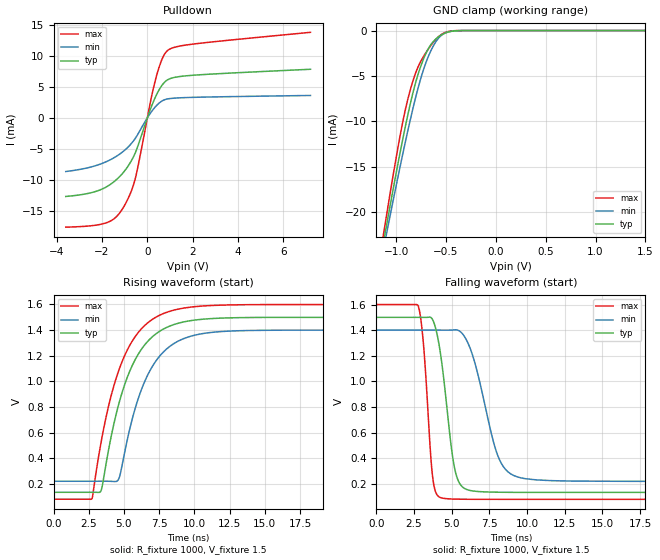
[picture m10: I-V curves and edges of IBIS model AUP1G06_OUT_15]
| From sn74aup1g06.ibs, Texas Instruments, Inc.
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[Model]   AUP1G06_OUT_15
Model_type  Open_drain
Enable   Active-Low
Vref =   1.5
Rref =   1E6
Cref =   30p
Vmeas =   0.75
| variable   typ   min   max
C_comp   1.68pF   1.45pF   1.95pF
| C_pulldown   2.10pF   1.70pF   2.55pF
| C_tri-state   1.68pF   1.45pF   1.95pF
[Temperature Range]   40   100   -40
| Ambient temperature   25   85   -40
[Voltage range]   1.5   1.4   1.6
[Pullup Reference]   1.5   1.5   1.5
[POWER Clamp Reference]   1.5   1.5   1.5
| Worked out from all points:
|   slope of the pulldown table from 0 to 0.225 V, typ, clamps not added: 101 ohm
|   GND clamp passes 1 mA (typ) near -0.61 V on its own axis
|   rising waveform, R_fixture 1000, V_fixture 1.5: 20-80 % time 2.29ns typ, 2.23ns min, 2.33ns max; typ from 0.133 V to 1.5 V
|   falling waveform, R_fixture 1000, V_fixture 1.5: 20-80 % time 824ps typ, 1.46ns min, 510ps max; typ from 1.5 V to 0.133 V
[GND Clamp]
| AUP1G06_OUT_15
|   Voltage   I(typ)   I(min)   I(max)
-3.6V     -193.5mA   -179.7mA   -210.2mA
-1.13V    -23.52mA   -24.27mA   -22.65mA
-1.105V   -21.98mA   -22.86mA   -20.94mA
-1.085V   -20.77mA   -21.75mA   -19.58mA
-950mV    -12.87mA   -14.45mA   -10.98mA
-850mV    -7.682mA   -9.442mA   -6.214mA
-790mV    -5.17mA    -6.745mA   -4.259mA
-720mV    -2.981mA   -4.114mA   -2.762mA
-650mV    -1.523mA   -2.183mA   -1.616mA
-580mV    -733.4uA   -904.6uA   -734uA
-390mV    -21.99uA   -24.69uA   -8.299uA
1.5V      133.6pA    590.3pA    26.39pA
[Pulldown]
| AUP1G06_OUT_15
|   Voltage   I(typ)   I(min)   I(max)
-3.6V     -12.64mA   -8.632mA   -17.58mA
-1.79V    -11.07mA   -7.008mA   -16.85mA
-1.38V    -9.983mA   -6.211mA   -15.95mA
-1.025V   -8.629mA   -5.274mA   -14.21mA
-725mV    -7.022mA   -4.203mA   -11.94mA
-525mV    -5.567mA   -3.253mA   -9.657mA
150mV     1.53mA     832.4uA    2.806mA
420mV     3.835mA    2.043mA    6.955mA
670mV     5.357mA    2.767mA    9.628mA
900mV     6.139mA    3.055mA    10.86mA
1.995V    6.857mA    3.303mA    11.87mA
7.2V      7.827mA    3.609mA    13.77mA
[Ramp]
| AUP1G06_OUT_15
| variable   typ   min   max
dV/dt_r   0.82/2.29E-09   0.71/2.23E-09   0.91/2.33E-09
dV/dt_f   0.82/8.28E-10   0.71/1.47E-09   0.91/5.12E-10
R_load = 1000
[Rising Waveform]
| AUP1G06_OUT_15
R_fixture =   1000
C_fixture =   0
L_fixture =   0
V_fixture =   1.5
V_fixture_min = 1.4
V_fixture_max = 1.6
|   Time   V(typ)   V(min)   V(max)
0s        133.1mV    219.3mV    79.08mV
2.73ns    133.2mV    219.3mV    83.54mV
3.395ns   152.2mV    219.5mV    534.8mV
4.555ns   790.3mV    224.5mV    1.06V
5.3ns     1.049V     574.7mV    1.258V
6.15ns    1.236V     908.6mV    1.399V
7.85ns    1.411V     1.234V     1.532V
9.555ns   1.471V     1.346V     1.577V
12.24ns   1.495V     1.391V     1.596V
34.99ns   1.5V       1.4V       1.6V
[Falling Waveform]
| AUP1G06_OUT_15
R_fixture =   1000
C_fixture =   0
L_fixture =   0
V_fixture =   1.5
V_fixture_min = 1.4
V_fixture_max = 1.6
|   Time   V(typ)   V(min)   V(max)
0s        1.5V       1.4V       1.6V
2.8ns     1.5V       1.4V       1.584V
3.15ns    1.5V       1.4V       1.266V
3.735ns   1.483V     1.4V       261.7mV
4.28ns    1.202V     1.4V       92.05mV
5.195ns   324.1mV    1.403V     80.97mV
6.1ns     152.1mV    1.296V     79.5mV
8.04ns    134.8mV    428.3mV    79.1mV
9.37ns    133.5mV    254mV      79.08mV
34.99ns   133.1mV    219.3mV    79.08mV
